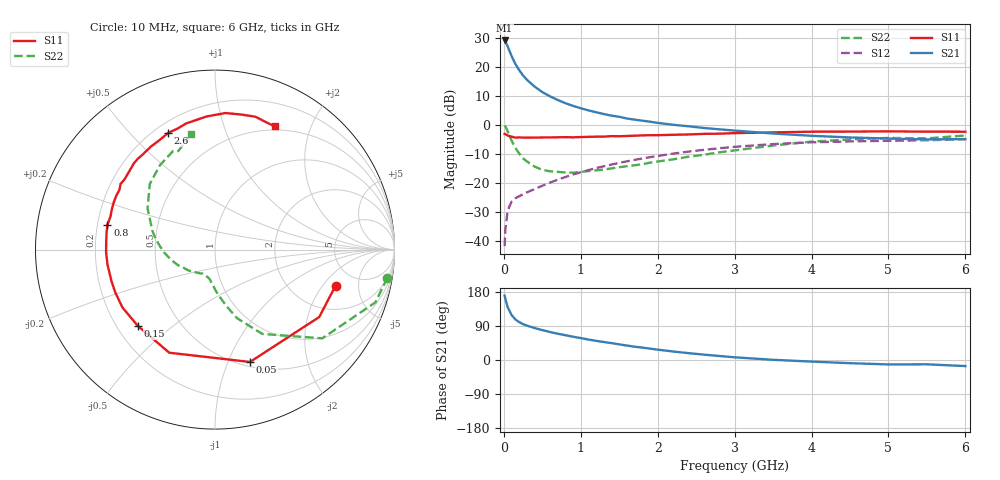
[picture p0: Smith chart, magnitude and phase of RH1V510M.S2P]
! SIEMENS Small Signal Semiconductors
! BFR106
! Si NPN RF Bipolar Junction Transistor in SOT23
! VCE = 1.5 V  IC = 10 mA
! Common Emitter S-Parameters:  August  1996
# GHz  S  MA  R  50
!  f  S11  S21  S12  S22
! GHz  MAG  ANG  MAG  ANG  MAG  ANG  MAG  ANG
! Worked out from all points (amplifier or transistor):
!   36 points, 10 MHz to 6 GHz, reference 50 ohm
!   highest |S21| = 29.0 dB at 10 MHz (marker M1)
!   |S21| within 3 dB of that: start of sweep to 64.29 MHz
!   unconditionally stable (mu >= 1): 465 MHz to 2.51 GHz; 4.316 GHz to end of sweep
!   at 250 MHz: K = 0.73, MSG = 20.4 dB, |S12| = -23.9 dB
!   at 1.4 GHz: K = 1.11, MAG = 6.4 dB, |S12| = -13.6 dB
!   at 6 GHz: K = 1.02, MAG = -0.9 dB, |S12| = -4.9 dB
!   S11 on the Smith chart (normalised r, x): 10 MHz: 3.42, -2.72; 50 MHz: 0.55, -1.20; 150 MHz: 0.29, -0.38; 800 MHz: 0.24, +0.11; 2.6 GHz: 0.25, +0.65; 6 GHz: 0.46, +1.50
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0.01  0.7012 -16.7  28.32 170.0  0.0082 82.0  0.9729 -9.3
0.02  0.6917 -32.9  27.28 161.5  0.016 76.0  0.941 -18.2
0.05  0.6557 -72.7  22.29 139.5  0.0337 58.9  0.7758 -39.6
0.1  0.6285 -113.9  15.38 118.8  0.0477 46.1  0.5387 -60.7
0.15  0.6045 -135.3  11.15 107.0  0.0547 42.5  0.4014 -72.2
0.2  0.6082 -147.9  8.741 99.9  0.0593 42.6  0.3203 -78.6
0.25  0.6049 -156.7  7.079 94.5  0.064 43.6  0.2653 -84.2
0.3  0.603 -163.1  5.966 90.7  0.069 45.6  0.2346 -88.3
0.4  0.6047 -172.1  4.553 84.4  0.0789 49.1  0.1916 -94.7
0.5  0.6069 -178.6  3.669 78.9  0.0897 52.0  0.1685 -99.8
0.6  0.6081 175.6  3.095 73.9  0.1018 54.1  0.1592 -104.2
0.7  0.6117 170.7  2.682 69.4  0.1139 55.7  0.1555 -109.0
0.8  0.6151 167.0  2.36 65.4  0.127 56.4  0.1519 -113.6
1.1  0.6226 154.8  1.777 54.0  0.1667 57.1  0.1607 -125.9
1.3  0.6278 148.0  1.536 47.4  0.1941 56.2  0.17 -133.9
1.6  0.6443 138.8  1.287 38.1  0.2361 54.0  0.1946 -145.6
2.2  0.6755 122.2  1.005 22.5  0.3202 46.6  0.2551 -168.5
2.6  0.7005 111.9  0.885 14.2  0.3718 40.5  0.3062 176.8
3.5  0.7435 93.5  0.71 0.5  0.4676 25.7  0.4413 148.4
4.5  0.7667 78.8  0.608 -8.4  0.5193 9.8  0.5614 123.1
5.5  0.7642 67.6  0.562 -11.4  0.5438 0.3  0.5861 110.4
6  0.7628 64.2  0.57 -16.0  0.5681 -6.8  0.6571 101.7
